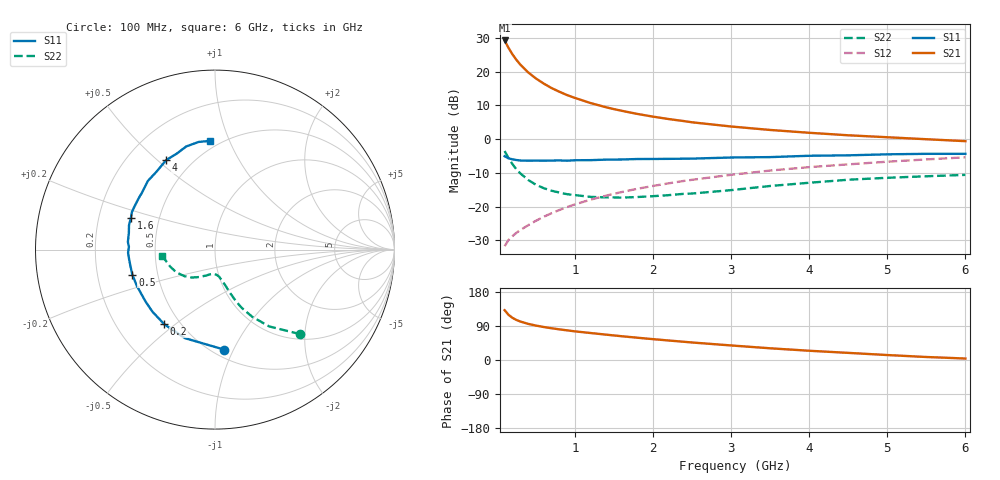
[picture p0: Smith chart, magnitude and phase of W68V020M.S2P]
! SIEMENS Small Signal Semiconductors
! BFR193W
! Si NPN RF Bipolar Junction Transistor in SOT323
! VCE = 8 V  IC = 20 mA
! Common Emitter S-Parameters:  September  1992
# GHz  S  MA  R  50
!  f  S11  S21  S12  S22
! GHz  MAG  ANG  MAG  ANG  MAG  ANG  MAG  ANG
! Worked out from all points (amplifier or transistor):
!   28 points, 100 MHz to 6 GHz, reference 50 ohm
!   highest |S21| = 29.3 dB at 100 MHz (marker M1)
!   |S21| within 3 dB of that: start of sweep to 171.1 MHz
!   unconditionally stable (mu >= 1): 818.1 MHz to 2.615 GHz
!   at 300 MHz: K = 0.74, MSG = 24.6 dB, |S12| = -27.0 dB
!   at 1.5 GHz: K = 1.04, MAG = 11.4 dB, |S12| = -16.2 dB
!   at 6 GHz: K = 0.91, MSG = 2.4 dB, |S12| = -5.4 dB
!   lowest NFmin = 1.40 dB at 450 MHz
!   S11 on the Smith chart (normalised r, x): 100 MHz: 0.57, -0.92; 200 MHz: 0.41, -0.46; 500 MHz: 0.36, -0.13; 1.6 GHz: 0.34, +0.16; 4 GHz: 0.36, +0.53; 6 GHz: 0.45, +0.85
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0.1  0.559 -84.9  29.14 131.4  0.0259 59.5  0.6681 -44.8
0.15  0.5211 -108.8  22.62 119.3  0.032 55.8  0.5239 -54.8
0.2  0.5028 -124.2  18.19 111.3  0.0364 54.8  0.4277 -61.0
0.25  0.4911 -135.2  15.07 105.8  0.0408 55.9  0.358 -65.3
0.3  0.4832 -143.2  12.84 101.6  0.0448 57.0  0.3123 -67.8
0.4  0.4801 -155.3  9.837 95.4  0.0528 59.8  0.2491 -71.3
0.5  0.4811 -163.2  7.969 90.9  0.0616 62.0  0.2117 -73.5
0.6  0.4802 -169.4  6.692 87.1  0.0706 63.7  0.1879 -76.1
0.7  0.4816 -173.8  5.747 83.8  0.0797 65.1  0.1722 -77.7
0.8  0.4847 -178.0  5.064 80.9  0.089 65.8  0.162 -79.8
0.9  0.4799 178.1  4.513 78.2  0.0985 66.5  0.1528 -81.1
1  0.4872 175.0  4.095 75.6  0.1078 66.7  0.1482 -83.0
1.2  0.4889 169.0  3.438 71.2  0.1269 66.8  0.1395 -87.4
1.4  0.4978 164.3  2.974 66.9  0.1454 66.6  0.137 -91.3
1.6  0.5002 159.6  2.638 62.7  0.1646 66.0  0.1358 -95.3
2.2  0.511 147.6  1.99 51.5  0.2216 63.1  0.1479 -106.2
2.5  0.5151 142.5  1.781 46.2  0.2498 61.3  0.1563 -111.2
3.5  0.5424 127.1  1.371 30.9  0.3428 53.9  0.2023 -129.7
4  0.5678 118.7  1.245 24.4  0.385 49.6  0.2258 -139.0
4.5  0.5762 111.5  1.143 18.8  0.4233 45.7  0.2505 -149.8
5.5  0.6068 98.6  0.999 7.9  0.5015 37.6  0.2819 -167.7
6  0.6065 92.4  0.935 3.9  0.5384 33.2  0.2957 -173.2
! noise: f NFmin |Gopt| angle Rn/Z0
0.45  1.4  0.3  160  0.1
0.9  1.45  0.34  172  0.11
1.8  2.2  0.56  -148  0.2
